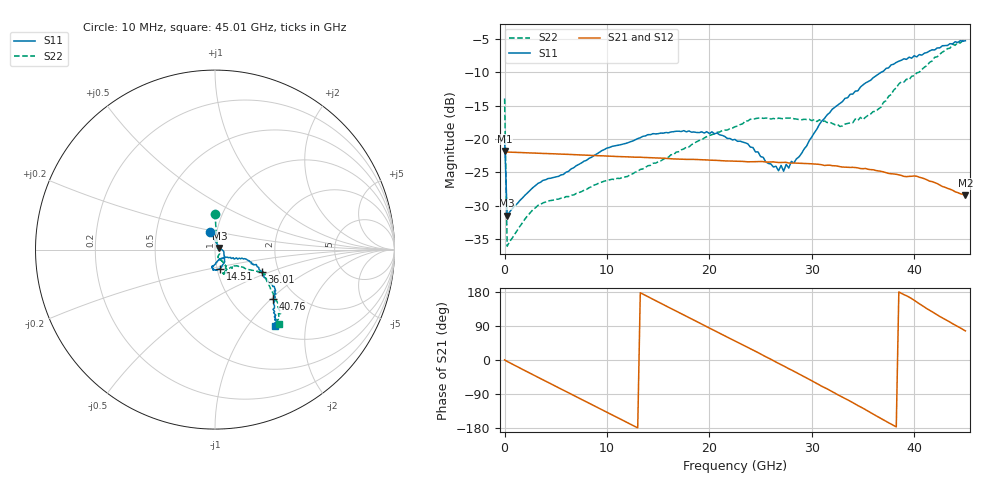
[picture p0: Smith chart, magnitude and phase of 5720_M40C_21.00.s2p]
! Device:  ADRF5720
! Description: 0.5dB LSB GaAs MMIC 6-bit Digital Attenuator
! Frequency:  0.000009 -  40 GHz
! Ports:
!	RF1	= Port 1
!	RF2	= Port 2
! Vdd:  3.3 Volt
! Vss:  -3.3 Volt
! Control:  0/3.3 Volt
! State:  21.00 dB attenuation
! Data:  The device was measured using G-S-G Probes on a matrix board.
!  Data was collected using an calibrated 4 port network analyzer.
!  The reference plane for this measurement is at the launchers.
! Note:  Analog Devices supplies this data as a sample of measured data
!  for this product.  Your particular data for this product may vary.
!  Data was taken at -40 degrees C.
!  Analog Devices reserves the right to change this data at anytime.
# GHZ S DB R 45.0
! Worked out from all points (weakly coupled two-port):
!   181 points, 10 MHz to 45.01 GHz, reference 45 ohm
!   highest |S21| = -21.77 dB at 10 MHz (marker M1); lowest = -28.4 dB at 45.01 GHz (marker M2)
!   lowest |S11| = -31.5 dB at 260 MHz (marker M3), VSWR 1.05, Z = 47.3 + j0.895 ohm
!   |S11| at or under -10 dB: start of sweep to 36.81 GHz
!   |S22| runs from -36.0 to -5.3 dB; largest |S21 - S12| = 0.00034
!   S11 on the Smith chart (normalised r, x): 10 MHz: 0.93, +0.18; 14.51 GHz: 1.04, -0.22; 36.01 GHz: 1.63, -0.44; 40.76 GHz: 1.54, -1.03; 45.01 GHz: 1.13, -1.37
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0.01  -19.96 106.7  -21.77 0.3  -21.80 0.3  -13.94 90.1
0.26  -31.46 20.7  -21.95 -3.8  -21.97 -3.8  -36.03 31.2
3.26  -26.65 -8.8  -22.13 -45.5  -22.15 -45.5  -29.94 -32.5
7.76  -23.32 -39.4  -22.40 -107.2  -22.42 -107.2  -27.67 -65.6
10.01  -21.35 -51.3  -22.55 -138.0  -22.57 -138.0  -26.20 -68.0
14.51  -19.20 -73.9  -22.81 160.1  -22.83 160.0  -23.63 -62.2
15.26  -19.12 -77.3  -22.85 149.6  -22.87 149.6  -23.27 -60.5
20.26  -18.92 -95.5  -23.17 80.9  -23.19 80.8  -19.35 -57.4
22.76  -20.35 -100.7  -23.33 46.7  -23.35 46.6  -18.06 -62.7
24.01  -21.21 -93.3  -23.41 29.9  -23.43 29.8  -17.04 -64.2
27.26  -24.82 -60.2  -23.51 -15.7  -23.53 -15.8  -16.98 -68.3
27.51  -23.80 -53.0  -23.49 -19.4  -23.51 -19.5  -16.86 -69.6
27.76  -24.34 -50.3  -23.59 -23.0  -23.62 -23.1  -16.88 -68.4
28.76  -22.67 -35.6  -23.62 -36.9  -23.64 -37.1  -17.10 -70.5
30.26  -19.07 -24.1  -23.74 -58.4  -23.76 -58.5  -17.08 -69.8
32.76  -14.66 -17.3  -24.14 -94.6  -24.16 -94.7  -18.13 -59.0
36.01  -10.83 -25.2  -24.60 -142.8  -24.63 -142.9  -15.89 -35.7
37.76  -8.92 -31.6  -25.20 -169.1  -25.23 -169.2  -13.35 -30.9
38.76  -8.22 -31.9  -25.45 176.0  -25.47 175.8  -11.44 -27.4
40.76  -7.45 -40.4  -25.82 144.2  -25.85 144.0  -9.59 -29.6
43.76  -5.78 -48.8  -27.66 95.8  -27.69 95.5  -5.83 -44.3
45.01  -5.30 -51.9  -28.42 76.8  -28.42 76.7  -5.26 -49.5
